FUNCTION "DIVE" : VOID
TITLE =
VERSION : 0.1


VAR_TEMP
  zero : BOOL ;
END_VAR
BEGIN
NETWORK
TITLE =Produzione in corso
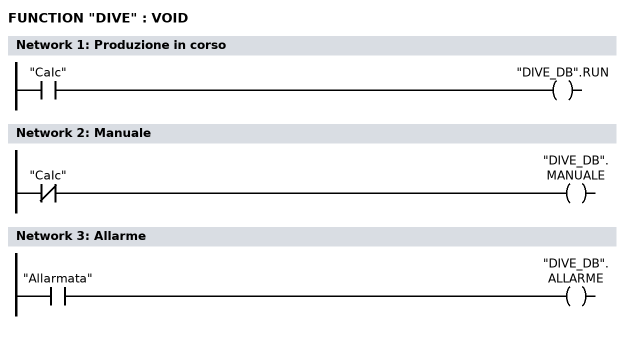
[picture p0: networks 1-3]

      U     "CaIc";
      =     "DIVE_DB".RUN;
NETWORK
TITLE =Manuale

      UN    "CaIc";
      =     "DIVE_DB".MANUALE;
NETWORK
TITLE =Allarme

      U     "Allarmata";
      =     "DIVE_DB".ALLARME;
NETWORK
TITLE =Bit sempre a zero

      CLR   ;
      =     "ALWAYS_0";
      U     "ALWAYS_0";
      =     #zero;
NETWORK
TITLE =Mancato Carico
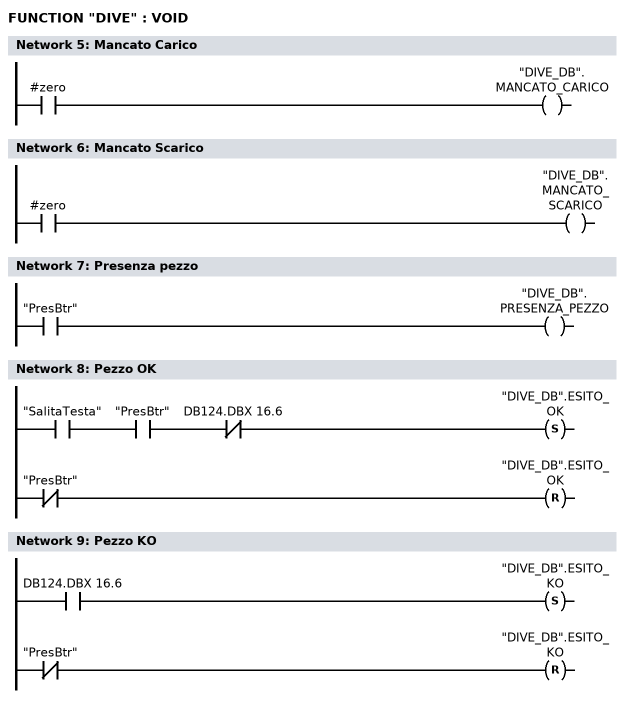
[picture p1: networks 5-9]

      U     #zero;
      =     "DIVE_DB".MANCATO_CARICO;
NETWORK
TITLE =Mancato Scarico

      U     #zero;
      =     "DIVE_DB".MANCATO_SCARICO;
NETWORK
TITLE =Presenza pezzo

      U     "PresBtr";
      =     "DIVE_DB".PRESENZA_PEZZO;
NETWORK
TITLE =Pezzo OK

      U     "SalitaTesta";
      U     "PresBtr";
      UN    DB124.DBX   16.6;
      S     "DIVE_DB".ESITO_OK;
      UN    "PresBtr";
      R     "DIVE_DB".ESITO_OK;
      NOP   0;
NETWORK
TITLE =Pezzo KO

      U     DB124.DBX   16.6;
      S     "DIVE_DB".ESITO_KO;
      UN    "PresBtr";
      R     "DIVE_DB".ESITO_KO;
      NOP   0;
NETWORK
TITLE =Fine Lavoro

      U(    ;
      U(    ;
      O     "SalitaTesta";
      O     DB124.DBX   16.6;
      )     ;
      S     M    254.3;
      UN    "PresBtr";
      R     M    254.3;
      U     M    254.3;
      )     ;
      L     S5T#500MS;
      SE    T     15;
      NOP   0;
      NOP   0;
      NOP   0;
      U     T     15;
      =     "DIVE_DB".FINE_LAVORO;
NETWORK
TITLE =Inizio Pallet
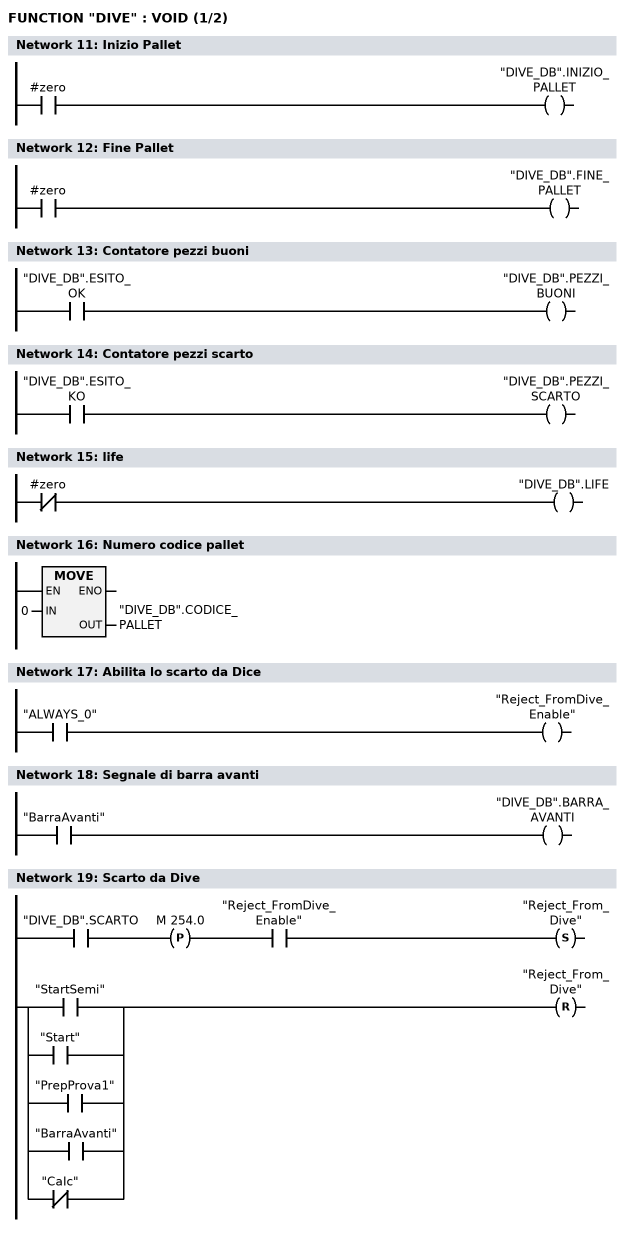
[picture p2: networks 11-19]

      U     #zero;
      =     "DIVE_DB".INIZIO_PALLET;
NETWORK
TITLE =Fine Pallet

      U     #zero;
      =     "DIVE_DB".FINE_PALLET;
NETWORK
TITLE =Contatore pezzi buoni

      U     "DIVE_DB".ESITO_OK;
      =     "DIVE_DB".PEZZI_BUONI;
NETWORK
TITLE =Contatore pezzi scarto

      U     "DIVE_DB".ESITO_KO;
      =     "DIVE_DB".PEZZI_SCARTO;
NETWORK
TITLE =life

      UN    #zero;
      =     "DIVE_DB".LIFE;
NETWORK
TITLE =Numero codice pallet

      L     0;
      T     "DIVE_DB".CODICE_PALLET;
      NOP   0;
NETWORK
TITLE =Abilita lo scarto da Dice

      U     "ALWAYS_0";
      =     "Reject_FromDive_Enable";
NETWORK
TITLE =Segnale di barra avanti

      U     "BarraAvanti";
      =     "DIVE_DB".BARRA_AVANTI;
NETWORK
TITLE =Scarto da Dive

      U     "DIVE_DB".SCARTO;
      FP    M    254.0;
      U     "Reject_FromDive_Enable";
      S     "Reject_From_Dive";
      U(    ;
      O     "StartSemi";
      O     "Start";
      O     "PrepProva1";
      O     "BarraAvanti";
      ON    "CaIc";
      )     ;
      R     "Reject_From_Dive";
      NOP   0;
NETWORK
TITLE =Pulsante di reset per scarto da tracciabilità
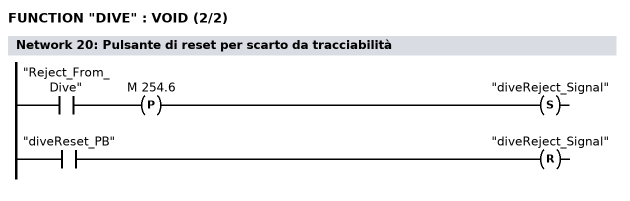
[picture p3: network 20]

      U     "Reject_From_Dive";
      FP    M    254.6;
      S     "diveReject_Signal";
      U     "diveReset_PB";
      R     "diveReject_Signal";
      NOP   0;
END_FUNCTION

